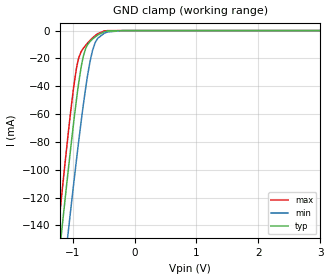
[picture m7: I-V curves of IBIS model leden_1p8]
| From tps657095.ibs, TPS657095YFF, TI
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|   leden_1p8 Model
[Model]   leden_1p8
Model_type   Input
Vinl = 0.4
Vinh = 1.2
|   typ   min   max
|   (nom PVT)   (fast PVT)   (slow PVT)
C_comp   1.720e-12   1.684e-12   1.794e-12
| Where nom  PVT is Nominal Process, 1.8V, 27C
|   Fast PVT is Strong Process,  2V, -40C
|   Slow PVT is Weak Process,   1.6V, 125C
[Voltage Range]   1.8   1.6   2
|Junction Temperature
[Temperature Range]   27   125   -40
[Power Clamp Reference]   1.8   1.6   2
[GND Clamp Reference]   0   0   0
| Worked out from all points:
|   GND clamp passes 1 mA (typ) near -0.50 V on its own axis
[GND Clamp]
|   Voltage   I(typ)   I(min)   I(max)
-1.8V     -422.3mA   -455.9mA   -406.2mA
-1.422V   -251.6mA   -291.6mA   -229.5mA
-1.202V   -155.5mA   -198.7mA   -130.1mA
-1.17V    -141.9mA   -185.5mA   -116.2mA
-1.066V   -98.72mA   -143.1mA   -72.19mA
-936mV    -49.29mA   -92.61mA   -26.9mA
-898mV    -36.71mA   -78.52mA   -19.35mA
-827.2mV  -18.64mA   -53.68mA   -12.8mA
-718.4mV  -7.854mA   -22.3mA    -7.102mA
-592.2mV  -3.171mA   -5.477mA   -2.21mA
-180mV    -147nA     -5.779uA   0A
3.6V      0A         0A         0A
[POWER Clamp]
|   Voltage   I(typ)   I(min)   I(max)
-1.8V     0A         0A         0A
0V        0A         0A         0A
3.6V      0A         0A         0A
